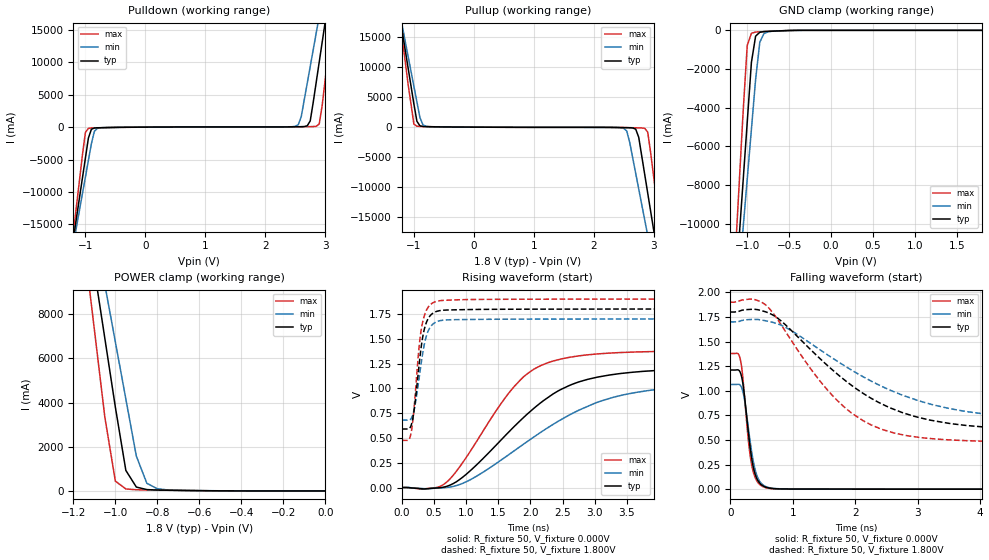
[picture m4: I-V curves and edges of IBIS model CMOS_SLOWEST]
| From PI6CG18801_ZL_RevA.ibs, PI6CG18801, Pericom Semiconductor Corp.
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|   Model REF_OUT
[Model]   CMOS_SLOWEST
Model_type Output
Vref=1.800V
Vmeas=900mV
| variable   typ   min   max
C_comp   1.500pF   1.470pF   1.530pF
[Voltage Range]   1.8000V   1.7000V   1.9000V
[POWER Clamp Reference]   1.8000V   1.7000V   1.9000V
[GND Clamp Reference]   0.0000V   0.0000V   0.0000V
[Pullup Reference]   1.8000V   1.7000V   1.9000V
[Pulldown Reference]   0.0000V   0.0000V   0.0000V
[Temperature Range]   25   85   -40
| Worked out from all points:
|   slope of the pulldown table from 0 to 0.27 V, typ, clamps not added: 17.5 ohm
|   slope of the pullup table from 0 to 0.27 V, typ, clamps not added: 20 ohm
|   GND clamp passes 1 mA (typ) near -0.37 V on its own axis
|   POWER clamp passes 1 mA (typ) near -0.40 V on its own axis
|   falling waveform, R_fixture 50, V_fixture 0.000V: 20-80 % time 139ps typ, 151ps min, 129ps max; typ from 1.21 V to 0 V
|   rising waveform, R_fixture 50, V_fixture 0.000V: 20-80 % time 1.23ns typ, 1.61ns min, 901ps max; typ from 0 V to 1.21 V
|   falling waveform, R_fixture 50, V_fixture 1.800V: 20-80 % time 1.48ns typ, 1.84ns min, 1.1ns max; typ from 1.8 V to 0.59 V
|   rising waveform, R_fixture 50, V_fixture 1.800V: 20-80 % time 135ps typ, 149ps min, 124ps max; typ from 0.59 V to 1.8 V
[GND Clamp]
| Voltage   I(typ)   I(min)   I(max)
-1.8V     -54.4A     -49.03A    -63.81A
-1.15V    -14.07A    -15.45A    -12.25A
-1.1V     -10.96A    -12.87A    -8.279A
-1.05V    -7.861A    -10.28A    -4.312A
-1V       -4.759A    -7.7A      -788.1mA
-950mV    -1.657A    -5.118A    -151.5mA
-900mV    -301.5mA   -2.536A    -89.47mA
-850mV    -99.76mA   -611.5mA   -76.41mA
-800mV    -65.24mA   -165.8mA   -67.68mA
-750mV    -53.48mA   -71.59mA   -57.6mA
-350mV    -497uA     -1.239mA   -102.1uA
1.8V      15.02uA    16.41uA    13.92uA
[Power Clamp]
| Voltage   I(typ)   I(min)   I(max)
-1.8V     53.54A     48.18A     62.95A
-1.15V    13.11A     14.51A     11.28A
-1.1V     10.01A     11.92A     7.303A
-1.05V    6.898A     9.333A     3.331A
-1V       3.791A     6.746A     443mA
-950mV    927.4mA    4.16A      88.83mA
-900mV    174mA      1.575A     52.93mA
-850mV    60.63mA    346.7mA    44.07mA
-800mV    39.38mA    97.65mA    37.38mA
-750mV    30.86mA    43.26mA    30.27mA
-650mV    18.32mA    20.25mA    16.82mA
0V        15.02uA    14.96uA    14.69uA
[Pulldown]
| Voltage   I(typ)   I(min)   I(max)
-1.8V     -54.42A    -49.05A    -63.84A
-1.2V     -17.2A     -18.06A    -16.25A
-1V       -4.79A     -7.726A    -827.2mA
-950mV    -1.689A    -5.144A    -191.1mA
-750mV    -87.68mA   -99.6mA    -100.8mA
2.55V     59.88mA    370.4mA    52.99mA
2.75V     956.7mA    9.357A     80.67mA
2.85V     6.928A     14.53A     125.7mA
2.9V      10.03A     17.12A     480mA
3V        16.25A     22.3A      7.34A
3.1V      22.47A     27.48A     15.29A
3.6V      53.58A     53.39A     55.04A
[Pullup]
| Voltage   I(typ)   I(min)   I(max)
-1.8V     53.63A     48.25A     63.06A
-1.2V     16.29A     17.15A     15.33A
-1V       3.851A     6.797A     513.7mA
-950mV    984.1mA    4.208A     156.8mA
-800mV    86.58mA    137.9mA    94.43mA
2.5V      -78.71mA   -194.9mA   -67.08mA
2.7V      -336.9mA   -7.729A    -111.4mA
2.85V     -7.897A    -15.48A    -195.5mA
2.9V      -11A       -18.06A    -832.2mA
3V        -17.2A     -23.23A    -8.323A
3.1V      -23.41A    -28.39A    -16.26A
3.6V      -54.44A    -54.22A    -55.93A
[Falling Waveform]
R_fixture = 50
V_fixture = 0.000V
V_fixture_min = 0.000V
V_fixture_max = 0.000V
|   Time   V(typ)   V(min)   V(max)
0s        1.211V     1.064V     1.378V
120ps     1.212V     1.065V     1.377V
168ps     1.169V     1.047V     1.289V
192ps     1.102V     1.009V     1.174V
228ps     929.4mV    899.4mV    922.8mV
300ps     503.5mV    558.6mV    421.7mV
372ps     207.5mV    264.1mV    161mV
468ps     62.62mV    79.77mV    48.94mV
648ps     8.917mV    12.06mV    4.843mV
20ns      8.49uV     9.345uV    8.037uV
[Rising Waveform]
R_fixture = 50
V_fixture = 0.000V
V_fixture_min = 0.000V
V_fixture_max = 0.000V
|   Time   V(typ)   V(min)   V(max)
0s        8.493uV    9.345uV    8.028uV
650ps     3.75mV     -1.811mV   31.04mV
1ns       132.6mV    57.63mV    302mV
1.55ns    483.5mV    279.5mV    852.7mV
1.9ns     709.6mV    440mV      1.12V
2.4ns     961.6mV    654.7mV    1.283V
2.85ns    1.083V     806.5mV    1.335V
3.85ns    1.175V     978.9mV    1.37V
5.6ns     1.206V     1.048V     1.378V
20ns      1.211V     1.064V     1.378V
[Falling Waveform]
R_fixture = 50
V_fixture = 1.800V
V_fixture_min = 1.700V
V_fixture_max = 1.900V
|   Time   V(typ)   V(min)   V(max)
0s        1.8V       1.7V       1.9V
375ps     1.828V     1.725V     1.929V
562.5ps   1.802V     1.711V     1.873V
1.438ns   1.325V     1.415V     1.096V
1.937ns   1.056V     1.211V     774.5mV
2.437ns   861.5mV    1.04V      605.5mV
3.063ns   721.6mV    889.1mV    522.9mV
4.188ns   626.7mV    754.5mV    485.6mV
6ns       595.6mV    694.9mV    476.2mV
20ns      589.9mV    679.5mV    475mV
[Rising Waveform]
R_fixture = 50
V_fixture = 1.800V
V_fixture_min = 1.700V
V_fixture_max = 1.900V
|   Time   V(typ)   V(min)   V(max)
0s        589.9mV    679.5mV    475mV
110ps     592.6mV    679.9mV    485mV
150ps     639.5mV    701.7mV    574.1mV
200ps     829.6mV    815.2mV    881.8mV
270ps     1.252V     1.115V     1.434V
300ps     1.416V     1.253V     1.587V
340ps     1.572V     1.413V     1.712V
430ps     1.724V     1.606V     1.835V
610ps     1.785V     1.684V     1.885V
20ns      1.8V       1.7V       1.9V
[Ramp]
| variable   typ   min   max
dV/dt_r   0.72534V/1.2368n   0.63822V/1.6099n   0.82706V/899.00p
dV/dt_f   0.72594V/1.4813n   0.61218V/1.8315n   0.85490V/1.0966n
R_load = 50
